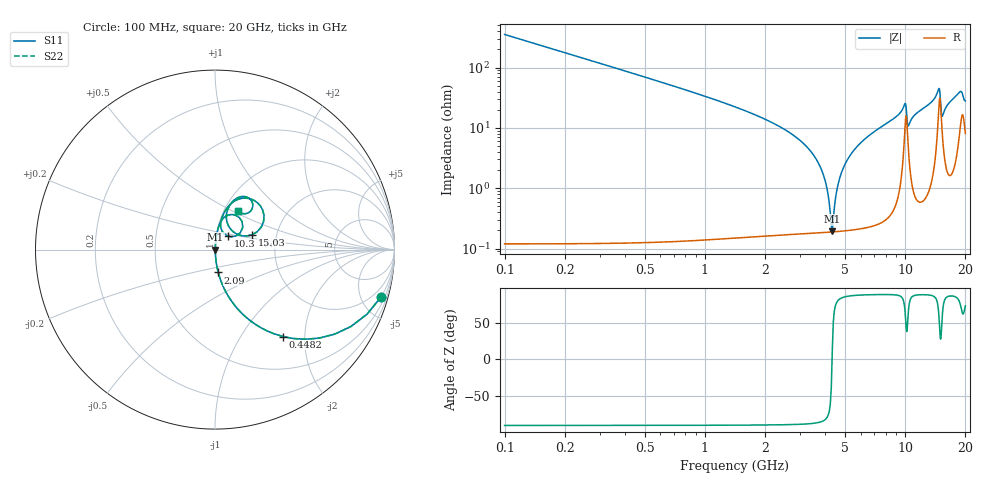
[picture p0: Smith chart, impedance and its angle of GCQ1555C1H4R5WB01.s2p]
!Murata Part Number: GCQ1555C1H4R5WB01
!These Parameters are Measured in Series Mode Connection
!Data Generated on Mar 13, 2026
!  o--ll--o
!Port1  Port2
!  o------o
!Operation Temp=25[degC], DC Bias Voltage=0[V]
!Freq. Start=100[MHz] Stop=20[GHz] 401[Steps]
# Hz S RI R 50
!Freq.(Hz) S11(Real) S11(Imag) S21(Real) S21(Imag) S12(Real) S12(Imag) S22(Real) S22(Imag)
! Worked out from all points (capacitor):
!   401 points, 100 MHz to 20 GHz, reference 50 ohm
!   read as one part in series: C = 4.5 pF near 199.5 MHz
!   lowest |Z| = 193 mohm at 4.329 GHz (marker M1)
!   series resonance near 4.319 GHz, so ESL is about 300 pH
!   S11 on the Smith chart (normalised r, x): 100 MHz: 1.00, -7.07; 448.2 MHz: 1.00, -1.56; 2.09 GHz: 1.00, -0.26; 10.3 GHz: 1.14, +0.17; 15.03 GHz: 1.49, +0.26; 20 GHz: 1.16, +0.54
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1e8  0.9258 -0.2619  0.0742 0.2619  0.0742 0.2619  0.9258 -0.2619
4.4825e8  0.3787 -0.4843  0.6213 0.4843  0.6213 0.4843  0.3787 -0.4843
9.4575e8  0.1134 -0.3152  0.8866 0.3152  0.8866 0.3152  0.1134 -0.3152
2.09e9  0.0181 -0.1272  0.9819 0.1272  0.9819 0.1272  0.0181 -0.1272
3.43325e9  0.00324 -0.038  0.9968 0.038  0.9968 0.038  0.00324 -0.038
3.93075e9  0.00208 -0.0155  0.9979 0.0155  0.9979 0.0155  0.00208 -0.0155
4.08e9  0.00194 -0.00938  0.9981 0.00938  0.9981 0.00938  0.00194 -0.00938
4.22925e9  0.00188 -0.00345  0.9981 0.00345  0.9981 0.00345  0.00188 -0.00345
4.32875e9  0.00188 0.000391  0.9981 -0.000391  0.9981 -0.000391  0.00188 0.000391
4.62725e9  0.00205 0.0114  0.998 -0.0114  0.998 -0.0114  0.00205 0.0114
5.02525e9  0.00261 0.0253  0.9974 -0.0253  0.9974 -0.0253  0.00261 0.0253
5.72175e9  0.00435 0.0476  0.9957 -0.0476  0.9957 -0.0476  0.00435 0.0476
6.7665e9  0.00853 0.0786  0.9915 -0.0786  0.9915 -0.0786  0.00853 0.0786
1.005e10  0.1512 0.1555  0.8488 -0.1555  0.8488 -0.1555  0.1512 0.1555
1.029875e10  0.0716 0.0758  0.9284 -0.0758  0.9284 -0.0758  0.0716 0.0758
1.338325e10  0.0716 0.2377  0.9284 -0.2377  0.9284 -0.2377  0.0716 0.2377
1.467675e10  0.236 0.2615  0.764 -0.2615  0.764 -0.2615  0.236 0.2615
1.5025e10  0.2069 0.0829  0.7931 -0.0829  0.7931 -0.0829  0.2069 0.0829
1.53235e10  0.0898 0.111  0.9102 -0.111  0.9102 -0.111  0.0898 0.111
1.67165e10  0.0794 0.2417  0.9206 -0.2417  0.9206 -0.2417  0.0794 0.2417
1.8806e10  0.1879 0.2873  0.8121 -0.2873  0.8121 -0.2873  0.1879 0.2873
2e10  0.1283 0.2163  0.8717 -0.2163  0.8717 -0.2163  0.1283 0.2163
